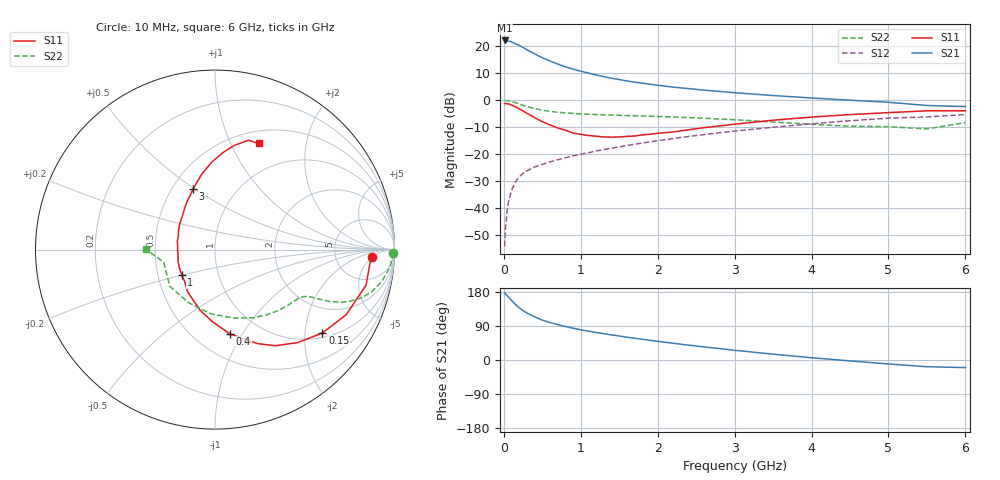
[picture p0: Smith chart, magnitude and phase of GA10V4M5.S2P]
! Infineon Technologies  Discrete & RF Semiconductors
! BF775
! Si NPN RF Bipolar Junction Transistor in SOT23
! VCE = 10 V  IC = 4.5 mA
! Common Emitter S-Parameters:  May  1996
# GHz  S  MA  R  50
!  f  S11  S21  S12  S22
! GHz  MAG  ANG  MAG  ANG  MAG  ANG  MAG  ANG
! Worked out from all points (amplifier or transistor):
!   36 points, 10 MHz to 6 GHz, reference 50 ohm
!   highest |S21| = 22.1 dB at 10 MHz (marker M1)
!   |S21| within 3 dB of that: start of sweep to 273.7 MHz
!   unconditionally stable (mu >= 1): 892.5 MHz to 2.981 GHz
!   at 250 MHz: K = 0.45, MSG = 23.3 dB, |S12| = -27.1 dB
!   at 1.4 GHz: K = 1.10, MAG = 11.0 dB, |S12| = -17.8 dB
!   at 6 GHz: K = 0.89, MSG = 1.5 dB, |S12| = -5.3 dB
!   S11 on the Smith chart (normalised r, x): 10 MHz: 13, -5; 150 MHz: 1.13, -2.47; 400 MHz: 0.73, -0.89; 1 GHz: 0.66, -0.20; 3 GHz: 0.63, +0.49; 6 GHz: 0.64, +1.28
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0.01  0.8735 -2.8  12.75 177.4  0.002 91.0  0.994 -1.1
0.02  0.8666 -5.3  12.45 174.8  0.0042 85.3  0.9881 -2.3
0.05  0.8644 -13.3  12.43 168.2  0.0113 83.9  0.9807 -5.7
0.1  0.816 -26.4  12.05 157.3  0.0216 76.0  0.9452 -10.9
0.15  0.7577 -37.8  11.08 146.8  0.0306 70.1  0.9032 -15.2
0.2  0.6939 -48.3  10.35 138.0  0.0383 66.4  0.8555 -18.4
0.25  0.632 -57.9  9.471 130.2  0.0444 62.6  0.8059 -20.9
0.3  0.5753 -65.6  8.555 124.1  0.0494 60.9  0.7654 -22.5
0.4  0.4777 -79.9  7.202 114.1  0.0583 58.1  0.7035 -24.3
0.5  0.4007 -92.3  6.11 105.3  0.0654 57.2  0.6547 -25.2
0.6  0.3491 -103.4  5.312 99.0  0.0725 56.9  0.6225 -25.8
0.8  0.2791 -123.4  4.151 88.4  0.0866 57.5  0.5834 -26.7
1  0.2333 -142.9  3.443 79.8  0.1002 58.3  0.5594 -27.9
1.1  0.2226 -152.9  3.174 76.2  0.1073 58.8  0.5504 -28.9
1.3  0.2089 -170.0  2.728 69.5  0.1223 59.2  0.5364 -30.7
1.6  0.215 167.7  2.272 60.2  0.1456 58.8  0.5206 -34.3
2.2  0.2594 134.7  1.746 44.2  0.1955 56.8  0.4908 -43.6
3  0.3599 109.8  1.377 25.6  0.2686 51.1  0.4362 -60.4
3.5  0.4273 99.9  1.221 15.4  0.3161 46.3  0.3954 -74.8
4.5  0.5421 85.4  1.001 -2.4  0.4184 34.7  0.3308 -116.2
5.5  0.6369 73.0  0.799 -17.7  0.4913 19.1  0.2946 -166.2
6  0.6391 67.7  0.764 -20.1  0.544 14.9  0.3859 179.6
